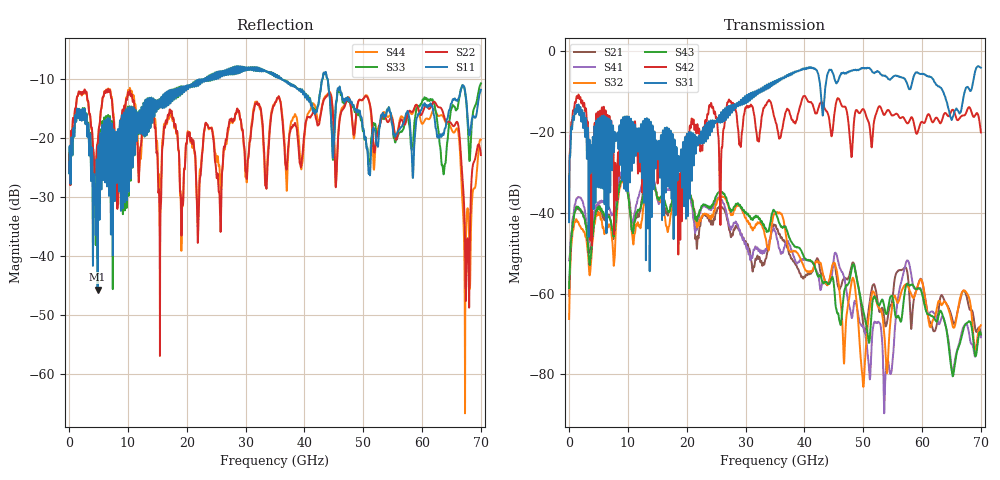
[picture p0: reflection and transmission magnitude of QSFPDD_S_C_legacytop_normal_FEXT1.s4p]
! AWR Design Environment (8415) Thu Dec 20 14:17:26 2018
! Document = 'CHANNEL TEST'
! nPorts: 4, nXvals: 7001
# HZ S DB R 50
!Freq DBS11 AngS11 DBS12 AngS12 DBS13 AngS13 DBS14 AngS14
!	DBS21 AngS21 DBS22 AngS22 DBS23 AngS23 DBS24 AngS24
!	DBS31 AngS31 DBS32 AngS32 DBS33 AngS33 DBS34 AngS34
!	DBS41 AngS41 DBS42 AngS42 DBS43 AngS43 DBS44 AngS44
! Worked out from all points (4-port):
!   7000 points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, 10 MHz to 70 GHz, reference 50 ohm
!   strongest paths, dB at 10 MHz, 17.51 GHz, 35.01 GHz, 52.51 GHz, 70 GHz:
!     S31: -42.3, -24.0, -7.5, -5.0, -4.0
!     S42: -41.2, -23.2, -16.9, -14.1, -20.1
!     S43: -58.6, -37.2, -39.6, -62.6, -70.1
!     S32: -66.3, -38.8, -40.0, -63.1, -67.8
!     S41: -51.7, -34.3, -44.5, -67.1, -70.8
!     S21: -60.5, -37.0, -43.1, -62.5, -70.3
!   lowest |S11| = -45.7 dB at 4.85 GHz (marker M1), VSWR 1.01, Z = 49.9 + j0.506 ohm
!   |S11| at or under -10 dB: start of sweep to 22.11 GHz; 36.16 GHz to 43.05 GHz (6.896 GHz wide, 17.4 % of centre); 43.97 GHz to end of sweep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
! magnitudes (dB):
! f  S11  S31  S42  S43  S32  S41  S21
! 10 MHz  -25.9  -42.3  -41.2  -58.6  -66.3  -51.7  -60.5
! 4.85 GHz  -45.7  -20.5  -16.5  -38.7  -39.7  -37.6  -38.2
! 35.82 GHz  -9.8  -7.2  -21.3  -42.7  -39.9  -49.0  -45.3
! 49.95 GHz  -18.4  -4.1  -14.3  -63.9  -82.1  -68.1  -67.2
! 65.95 GHz  -13.6  -14.4  -16.9  -74.4  -65.2  -74.1  -65.0
! 67.72 GHz  -16.0  -8.8  -14.3  -67.1  -60.1  -68.0  -61.7
! 70 GHz  -11.8  -4.0  -20.1  -70.1  -67.8  -70.8  -70.3
